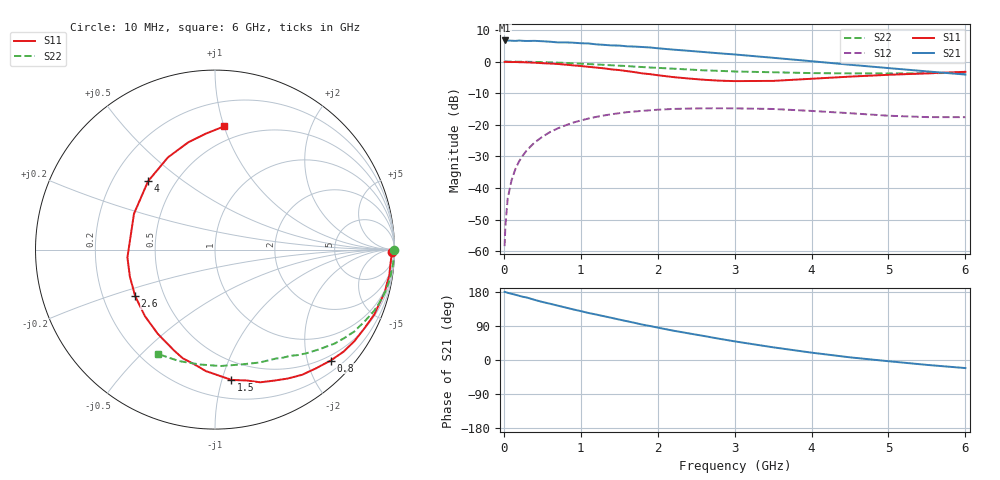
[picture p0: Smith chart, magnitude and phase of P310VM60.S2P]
! SIEMENS Small Signal Semiconductors
! BFP181
! Si NPN RF Bipolar Junction Transistor in SOT143
! VCE = 10 V  IC = 0.6 mA
! Common Emitter S-Parameters:  March  1996
# GHz  S  MA  R  50
!  f  S11  S21  S12  S22
! GHz  MAG  ANG  MAG  ANG  MAG  ANG  MAG  ANG
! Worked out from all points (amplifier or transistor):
!   36 points, 10 MHz to 6 GHz, reference 50 ohm
!   highest |S21| = 6.7 dB at 10 MHz (marker M1)
!   |S21| within 3 dB of that: start of sweep to 2.257 GHz
!   unconditionally stable (mu >= 1): 3.748 GHz to end of sweep
!   at 250 MHz: K = 0.08, MSG = 18.1 dB, |S12| = -29.7 dB
!   at 1.4 GHz: K = 0.43, MSG = 10.9 dB, |S12| = -16.7 dB
!   at 6 GHz: K = 1.39, MAG = 3.0 dB, |S12| = -17.6 dB
!   S11 on the Smith chart (normalised r, x): 10 MHz: open; 800 MHz: 0.40, -2.43; 1.5 GHz: 0.34, -1.07; 2.6 GHz: 0.34, -0.24; 4 GHz: 0.35, +0.38; 6 GHz: 0.38, +1.00
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0.01  0.9849 -0.7  2.153 179.6  0.0012 88.5  0.9993 -0.2
0.02  0.9942 -1.1  2.144 179.4  0.0025 81.1  0.9954 -0.5
0.05  0.983 -2.6  2.149 177.3  0.0068 90.0  0.9975 -1.4
0.1  0.9804 -5.5  2.133 174.8  0.0132 83.5  0.9968 -2.7
0.15  0.982 -8.4  2.118 172.2  0.0199 83.2  0.9958 -4.0
0.2  0.9764 -11.2  2.147 169.4  0.0266 82.4  0.9937 -5.4
0.3  0.9677 -16.6  2.112 164.8  0.0397 78.3  0.9896 -8.1
0.4  0.958 -22.2  2.123 158.7  0.0524 74.5  0.9849 -10.8
0.5  0.9409 -27.8  2.093 153.2  0.0643 70.1  0.9784 -13.5
0.8  0.893 -43.8  2.007 138.6  0.0977 59.0  0.9501 -21.0
1.1  0.8246 -60.6  1.931 124.1  0.1254 48.7  0.9114 -28.0
1.5  0.7318 -82.8  1.788 106.7  0.1523 36.4  0.8587 -36.3
1.8  0.649 -100.3  1.696 93.4  0.1659 28.5  0.8179 -41.7
1.9  0.6313 -106.6  1.668 89.7  0.1692 25.6  0.8041 -43.7
2.2  0.5675 -124.1  1.543 77.5  0.1777 18.6  0.7707 -48.5
2.6  0.5148 -149.8  1.412 63.4  0.1817 10.4  0.7251 -54.7
3  0.4899 -174.9  1.293 49.2  0.1815 2.7  0.6954 -60.8
3.5  0.4937 156.1  1.145 33.5  0.1775 -4.9  0.6762 -68.5
4  0.5334 134.3  1.011 19.4  0.1653 -10.5  0.6559 -77.4
4.5  0.5769 117.0  0.889 7.0  0.1522 -14.2  0.6494 -87.3
5.5  0.6494 94.2  0.698 -12.9  0.1321 -12.4  0.6527 -107.9
6  0.6879 85.9  0.622 -21.3  0.1317 -9.2  0.6628 -118.8
